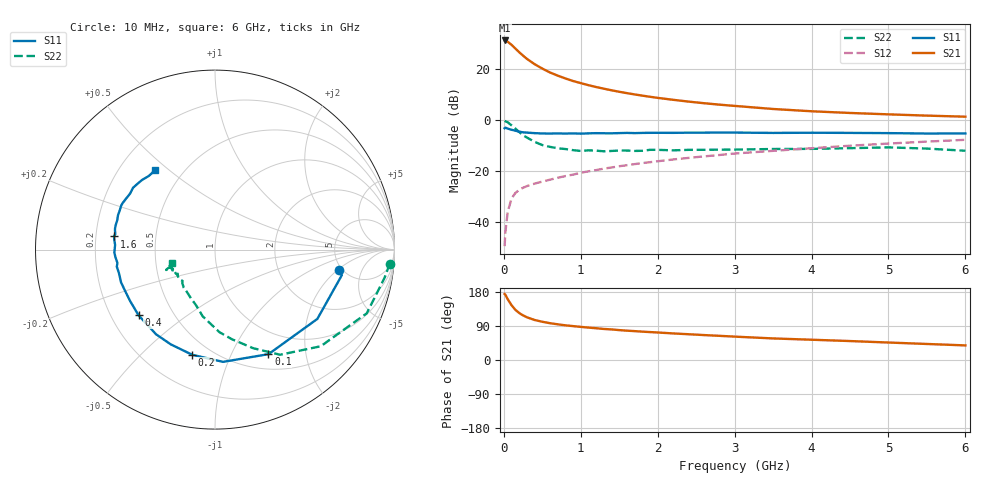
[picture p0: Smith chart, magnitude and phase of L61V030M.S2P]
!  INFINEON TECHNOLOGIES Small Signal Semiconductors
! BFR380L3 , Si-NPN RF-Transistor in TSLP-3-1
!  Vce=1 V,  Ic=30 mA
! Common Emitter S-Parameters:  07. March 2005
#  GHz  S  MA  R  50
! f  S11  S21  S12  S22
! GHz  Mag  Ang  Mag  Ang  Mag  Ang  Mag  Ang
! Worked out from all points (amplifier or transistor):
!   36 points, 10 MHz to 6 GHz, reference 50 ohm
!   highest |S21| = 31.4 dB at 10 MHz (marker M1)
!   |S21| within 3 dB of that: start of sweep to 144.4 MHz
!   unconditionally stable (mu >= 1): 1.625 GHz to 5.392 GHz
!   at 250 MHz: K = 0.42, MSG = 25.9 dB, |S12| = -26.4 dB
!   at 1.4 GHz: K = 0.98, MSG = 15.1 dB, |S12| = -18.5 dB
!   at 6 GHz: K = 0.99, MSG = 4.5 dB, |S12| = -7.6 dB
!   S11 on the Smith chart (normalised r, x): 10 MHz: 4.66, -2.10; 100 MHz: 0.69, -1.40; 200 MHz: 0.40, -0.73; 400 MHz: 0.32, -0.34; 1.6 GHz: 0.28, +0.06; 6 GHz: 0.35, +0.45
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0.01  0.699 -9.5  36.97 174.2  0.0034 78.6  0.9769 -4.6
0.02  0.7209 -11.4  36.51 172.2  0.0064 84.4  0.9579 -9.4
0.05  0.6887 -34.1  34.93 160.5  0.0159 75.9  0.9168 -22.8
0.1  0.6543 -62.9  30.37 144.6  0.0293 64.3  0.7983 -42.4
0.15  0.6271 -85.9  25.69 132.5  0.0376 55.8  0.6893 -58.2
0.2  0.5996 -102.2  21.68 123.9  0.0434 52.6  0.5901 -68.7
0.25  0.5827 -115.0  18.61 117.7  0.0476 49.8  0.5089 -79.2
0.3  0.5749 -124.8  16.09 112.7  0.0513 49.3  0.461 -86.9
0.4  0.5616 -139.3  12.65 105.6  0.0574 48.3  0.3782 -100.4
0.5  0.553 -148.8  10.37 100.9  0.0629 50.2  0.328 -108.7
0.6  0.5514 -155.7  8.699 97.1  0.0686 52.1  0.3022 -116.4
0.7  0.5543 -160.8  7.547 94.2  0.0747 53.8  0.2833 -123.5
0.9  0.5552 -170.1  5.918 89.4  0.0862 56.7  0.2602 -134.4
1.1  0.556 -175.5  4.9 85.5  0.1 58.5  0.2582 -139.7
1.3  0.5582 178.8  4.185 81.9  0.113 59.9  0.2471 -147.1
1.6  0.5675 172.6  3.421 77.4  0.1319 61.0  0.2557 -152.6
2.2  0.5687 163.3  2.532 70.1  0.1709 62.3  0.2579 -155.0
2.8  0.5774 154.8  2.036 63.8  0.2091 62.5  0.2661 -159.7
3.5  0.5668 146.5  1.672 56.9  0.2523 60.7  0.2742 -158.7
4.5  0.5674 140.2  1.397 50.0  0.3178 58.8  0.2847 -158.2
5.5  0.5515 131.9  1.239 42.3  0.3827 54.7  0.2794 -158.8
6  0.5544 126.9  1.181 38.5  0.4156 52.4  0.2533 -163.0
